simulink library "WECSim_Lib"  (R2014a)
settings: Solver=ode45  StartTime=0.0  StopTime=10.0  RelTol=1e-3
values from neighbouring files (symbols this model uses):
  geometry = 'NOT DEFINED'    [bodyClass.m]
  m = plot(Rel.WEC_Sim_org.time(find(Rel.WEC_Sim_org.time==350):end),     Rel.WEC_Sim_org.heave(find(Rel.WEC_Sim_org.time==350):end),'r-',     Rel.WEC_Sim_new.time(find(Rel.WEC_Sim_new.time==350):end),     Rel.WEC_Sim_new.heave(find(Rel.WEC_Sim_new.time==350):end),'k-')    [runTestCase.m]
  simu = simulationClass    [wecSim.m]
  waves = waveClass(waves.type,0,0,simu,'Imported',waves.randPreDefined,waves.spectrumDataFile)    [waveSetup.m]
undefined symbols (not defined in the file or in its folder): body, constraint, deg, flap, kg, N, pto, rad, s, X, Y, Z
libraries: nesl_utility x41, sm_lib x30
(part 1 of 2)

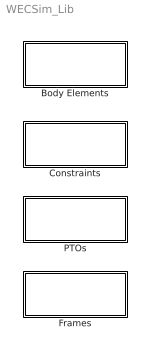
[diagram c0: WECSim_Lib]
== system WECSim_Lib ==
  Body Elements : Subsystem
  Constraints : Subsystem
  Frames : Subsystem
  PTOs : Subsystem

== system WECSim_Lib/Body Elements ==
  Rigid Body : Subsystem

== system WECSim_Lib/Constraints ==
  Fixed : Subsystem
  Floating : Subsystem
  Heave : Subsystem
  Pitch : Subsystem
  Surge : Subsystem

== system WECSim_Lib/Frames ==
  Global Reference Frame : Subsystem

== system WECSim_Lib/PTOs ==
  Rotational PTO (Local RY) : Subsystem
  Translational PTO (Local X) : Subsystem
  Translational PTO (Local Z) : Subsystem

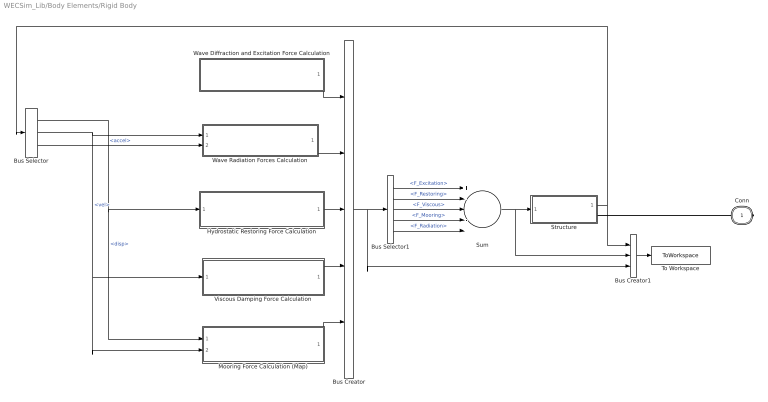
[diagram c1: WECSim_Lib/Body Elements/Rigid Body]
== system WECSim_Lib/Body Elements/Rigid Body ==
  Bus Creator : BusCreator  Inputs=5
  Bus Creator1 : BusCreator  Inputs=3
  Bus Selector : BusSelector  OutputSignals=disp,vel,accel
  Bus Selector1 : BusSelector  OutputSignals=F_Excitation,F_Restoring,F_Viscous,F_Mooring,F_Radiation
  Hydrostatic Restoring Force Calculation : Subsystem
  Mooring Force Calculation (Map) : Subsystem
  Structure : Subsystem
  Sum : Sum  Inputs=+----
  To Workspace : ToWorkspace  VariableName=Flap_out  SaveFormat=Structure With Time  SampleTime=-1
  Viscous Damping Force Calculation : Subsystem
  Wave Diffraction and Excitation Force Calculation : Subsystem
  Wave Radiation Forces Calculation : Subsystem
  Conn : PMIOPort  Port=1  Side=Right
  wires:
  Sum/1 -> Bus Creator1/2, Structure/1(F_vector)
  Bus Selector/1 -> Mooring Force Calculation (Map)/1(Displacement), Hydrostatic Restoring Force Calculation/1(Displacement)  "<disp>"
  Bus Selector/2 -> Mooring Force Calculation (Map)/2(Velocity), Viscous Damping Force Calculation/1(Velocity), Wave Radiation Forces Calculation/1(Velocity)  "<vel>"
  Structure/1(Response) -> Bus Selector/1, Bus Creator1/1
  Bus Creator/1 -> Bus Creator1/3, Bus Selector1/1
  Bus Creator1/1 -> To Workspace/1
  Bus Selector/3 -> Wave Radiation Forces Calculation/2(Acceleration)  "<accel>"
  Mooring Force Calculation (Map)/1(F_Mooring) -> Bus Creator/5
  Viscous Damping Force Calculation/1(F_Viscous) -> Bus Creator/4
  Hydrostatic Restoring Force Calculation/1(F_Restoring) -> Bus Creator/3
  Wave Radiation Forces Calculation/1(F_Radiation) -> Bus Creator/2
  Wave Diffraction and Excitation Force Calculation/1(F_Excitation) -> Bus Creator/1
  Bus Selector1/1 -> Sum/1  "<F_Excitation>"
  Bus Selector1/2 -> Sum/2  "<F_Restoring>"
  Bus Selector1/3 -> Sum/3  "<F_Viscous>"
  Bus Selector1/4 -> Sum/4  "<F_Mooring>"
  Bus Selector1/5 -> Sum/5  "<F_Radiation>"
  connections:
  Structure/RConn1 -- Conn/RConn1

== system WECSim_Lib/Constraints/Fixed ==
  Mux : Mux  Inputs=2
  PSS : nesl_utility/PS-Simulink Converter  PhysicalDomain=network_engine_domain  SubClassName=ps_output  LeftPortType=input  RightPortType=output  PseudoPeriodic=off  Frequencies=[]  Unit=1  AffineConversion=off
  PSS1 : nesl_utility/PS-Simulink Converter  PhysicalDomain=network_engine_domain  SubClassName=ps_output  LeftPortType=input  RightPortType=output  PseudoPeriodic=off  Frequencies=[]  Unit=1  AffineConversion=off
  Weld Joint : sm_lib/Joints/Weld Joint  SenseConstraintForce=on  SenseConstraintForceX=off  SenseConstraintForceY=off  SenseConstraintForceZ=off  SenseConstraintTorque=on  SenseConstraintTorqueX=off  SenseConstraintTorqueY=off  SenseConstraintTorqueZ=off  SenseTotalForce=off  SenseTotalForceX=off  SenseTotalForceY=off  SenseTotalForceZ=off  SenseTotalTorque=off  SenseTotalTorqueX=off  SenseTotalTorqueY=off  SenseTotalTorqueZ=off  CompositeWrenchDir=FollowerOnBase  CompositeWrenchFrame=BaseFrame  BlockFunction=simmechanics.library.joints.weld_joint
  output : ToWorkspace  VariableName=constraint1_out  SaveFormat=Structure With Time  SampleTime=-1
  B : PMIOPort  Port=1  Side=Left
  F : PMIOPort  Port=2  Side=Right
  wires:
  PSS/1 -> Mux/1
  PSS1/1 -> Mux/2
  Mux/1 -> output/1  "Constraint Forces"
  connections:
  Weld Joint/LConn1 -- B/RConn1
  F/RConn1 -- Weld Joint/RConn1
  PSS1/LConn1 -- Weld Joint/RConn3
  PSS/LConn1 -- Weld Joint/RConn2

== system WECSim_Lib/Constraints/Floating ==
  Mux : Mux  Inputs=2
  PSS : nesl_utility/PS-Simulink Converter  PhysicalDomain=network_engine_domain  SubClassName=ps_output  LeftPortType=input  RightPortType=output  PseudoPeriodic=off  Frequencies=[]  Unit=1  AffineConversion=off
  PSS1 : nesl_utility/PS-Simulink Converter  PhysicalDomain=network_engine_domain  SubClassName=ps_output  LeftPortType=input  RightPortType=output  PseudoPeriodic=off  Frequencies=[]  Unit=1  AffineConversion=off
  Planar Joint : sm_lib/Joints/Planar Joint  SenseConstraintForce=on  SenseConstraintForceX=off  SenseConstraintForceY=off  SenseConstraintForceZ=off  SenseConstraintTorque=on  SenseConstraintTorqueX=off  SenseConstraintTorqueY=off  SenseConstraintTorqueZ=off  SenseTotalForce=off  SenseTotalForceX=off  SenseTotalForceY=off  SenseTotalForceZ=off  SenseTotalTorque=off  SenseTotalTorqueX=off  SenseTotalTorqueY=off  SenseTotalTorqueZ=off  CompositeWrenchDir=FollowerOnBase  CompositeWrenchFrame=BaseFrame  PxEquilibriumPosition=0  PxEquilibriumPositionUnits=m  PxSpringStiffness=0  PxSpringStiffnessUnits=N/m  PxDampingCoefficient=0  PxDampingCoefficientUnits=N/(m/s)  PxTorqueActuationMode=NoTorque  PxMotionActuationMode=ComputedMotion  PxSensePosition=off  PxSenseVelocity=off  PxSenseAcceleration=off  PxSenseTorqueForce=off  PxPositionTargetValue=0  PxPositionTargetValueUnits=m  PxPositionTargetSpecify=off  PxPositionTargetPriority=High  PxVelocityTargetValue=0  PxVelocityTargetValueUnits=m/s  PxVelocityTargetSpecify=off  PxVelocityTargetPriority=High  PyEquilibriumPosition=0  PyEquilibriumPositionUnits=m  PySpringStiffness=0  PySpringStiffnessUnits=N/m  PyDampingCoefficient=0  PyDampingCoefficientUnits=N/(m/s)  PyTorqueActuationMode=NoTorque  PyMotionActuationMode=ComputedMotion  PySensePosition=off  PySenseVelocity=off  PySenseAcceleration=off  PySenseTorqueForce=off  PyPositionTargetValue=0  PyPositionTargetValueUnits=m  PyPositionTargetSpecify=off  PyPositionTargetPriority=High  PyVelocityTargetValue=0  PyVelocityTargetValueUnits=m/s  PyVelocityTargetSpecify=off  PyVelocityTargetPriority=High  RzEquilibriumPosition=0  RzEquilibriumPositionUnits=deg  RzSpringStiffness=0  RzSpringStiffnessUnits=N*m/deg  RzDampingCoefficient=0  RzDampingCoefficientUnits=N*m/(deg/s)  RzTorqueActuationMode=NoTorque  RzMotionActuationMode=ComputedMotion  RzSensePosition=off  RzSenseVelocity=off  RzSenseAcceleration=off  RzSenseTorqueForce=off  RzPositionTargetValue=0  RzPositionTargetValueUnits=deg  RzPositionTargetSpecify=off  RzPositionTargetPriority=High  RzVelocityTargetValue=0  RzVelocityTargetValueUnits=deg/s  RzVelocityTargetSpecify=off  RzVelocityTargetPriority=High  BlockFunction=simmechanics.library.joints.planar_joint
  Rigid Transform : sm_lib/Frames and Transforms/Rigid Transform  TranslationMethod=Cartesian  TranslationLengthUnit=m  TranslationStandardAxis=+Z  TranslationStandardOffset=0  TranslationCartesianOffset=[0 0 0]  TranslationROffset=0  TranslationROffsetUnits=m  TranslationZOffset=0  TranslationZOffsetUnits=m  TranslationThetaOffset=0  TranslationThetaOffsetUnits=deg  RotationMethod=StandardAxis  RotationAngleUnits=deg  RotationStandardAxis=+X  RotationAngle=90  RotationArbitraryAxis=[0 0 1]  FollAlignAxisA=+X  BaseAlignAxisA=+Y  FollAlignAxisB=+Y  BaseAlignAxisB=+Z  BlockFunction=simmechanics.library.frames_transforms.rigid_transform
  Rigid Transform1 : sm_lib/Frames and Transforms/Rigid Transform  TranslationMethod=Cartesian  TranslationLengthUnit=m  TranslationStandardAxis=+Z  TranslationStandardOffset=0  TranslationCartesianOffset=[0 0 0]  TranslationROffset=0  TranslationROffsetUnits=m  TranslationZOffset=0  TranslationZOffsetUnits=m  TranslationThetaOffset=0  TranslationThetaOffsetUnits=deg  RotationMethod=StandardAxis  RotationAngleUnits=deg  RotationStandardAxis=+X  RotationAngle=90  RotationArbitraryAxis=[0 0 1]  FollAlignAxisA=+X  BaseAlignAxisA=+Y  FollAlignAxisB=+Y  BaseAlignAxisB=+Z  BlockFunction=simmechanics.library.frames_transforms.rigid_transform
  output : ToWorkspace  VariableName=constraint1_out  SaveFormat=Structure With Time  SampleTime=-1
  B : PMIOPort  Port=1  Side=Left
  F : PMIOPort  Port=2  Side=Right
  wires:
  PSS/1 -> Mux/1
  PSS1/1 -> Mux/2
  Mux/1 -> output/1  "Constraint Forces"
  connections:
  Rigid Transform1/LConn1 -- F/RConn1
  Planar Joint/RConn1 -- Rigid Transform1/RConn1
  Rigid Transform/RConn1 -- Planar Joint/LConn1
  B/RConn1 -- Rigid Transform/LConn1
  PSS/LConn1 -- Planar Joint/RConn2
  PSS1/LConn1 -- Planar Joint/RConn3

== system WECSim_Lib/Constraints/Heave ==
  Mux : Mux  Inputs=2
  PSS : nesl_utility/PS-Simulink Converter  PhysicalDomain=network_engine_domain  SubClassName=ps_output  LeftPortType=input  RightPortType=output  PseudoPeriodic=off  Frequencies=[]  Unit=1  AffineConversion=off
  PSS1 : nesl_utility/PS-Simulink Converter  PhysicalDomain=network_engine_domain  SubClassName=ps_output  LeftPortType=input  RightPortType=output  PseudoPeriodic=off  Frequencies=[]  Unit=1  AffineConversion=off
  Translational Constraint (Prismatic Joint) : sm_lib/Joints/Prismatic Joint  SenseConstraintForce=on  SenseConstraintForceX=off  SenseConstraintForceY=off  SenseConstraintForceZ=off  SenseConstraintTorque=on  SenseConstraintTorqueX=off  SenseConstraintTorqueY=off  SenseConstraintTorqueZ=off  SenseTotalForce=off  SenseTotalForceX=off  SenseTotalForceY=off  SenseTotalForceZ=off  SenseTotalTorque=off  SenseTotalTorqueX=off  SenseTotalTorqueY=off  SenseTotalTorqueZ=off  CompositeWrenchDir=FollowerOnBase  CompositeWrenchFrame=BaseFrame  EquilibriumPosition=0  EquilibriumPositionUnits=m  SpringStiffness=0  SpringStiffnessUnits=N/m  DampingCoefficient=0  DampingCoefficientUnits=N/(m/s)  TorqueActuationMode=NoTorque  MotionActuationMode=ComputedMotion  SensePosition=off  SenseVelocity=off  SenseAcceleration=off  SenseTorqueForce=off  PositionTargetValue=0  PositionTargetValueUnits=m  PositionTargetSpecify=off  PositionTargetPriority=High  VelocityTargetValue=0  VelocityTargetValueUnits=m/s  VelocityTargetSpecify=off  VelocityTargetPriority=High  BlockFunction=simmechanics.library.joints.prismatic_joint
  output : ToWorkspace  VariableName=constraint1_out  SaveFormat=Structure With Time  SampleTime=-1
  F : PMIOPort  Port=1  Side=Right
  B : PMIOPort  Port=2  Side=Left
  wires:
  PSS/1 -> Mux/1
  PSS1/1 -> Mux/2
  Mux/1 -> output/1  "Constraint Forces"
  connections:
  B/RConn1 -- Translational Constraint (Prismatic Joint)/LConn1
  Translational Constraint (Prismatic Joint)/RConn1 -- F/RConn1
  PSS/LConn1 -- Translational Constraint (Prismatic Joint)/RConn2
  PSS1/LConn1 -- Translational Constraint (Prismatic Joint)/RConn3

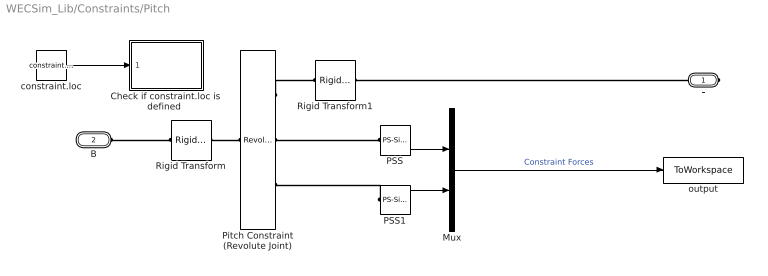
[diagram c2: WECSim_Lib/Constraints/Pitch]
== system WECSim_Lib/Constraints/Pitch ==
  "Check if constraint.loc is defined " : MATLAB Function  TreatAsAtomicUnit=on
  Mux : Mux  Inputs=2
  PSS : nesl_utility/PS-Simulink Converter  PhysicalDomain=network_engine_domain  SubClassName=ps_output  LeftPortType=input  RightPortType=output  PseudoPeriodic=off  Frequencies=[]  Unit=1  AffineConversion=off
  PSS1 : nesl_utility/PS-Simulink Converter  PhysicalDomain=network_engine_domain  SubClassName=ps_output  LeftPortType=input  RightPortType=output  PseudoPeriodic=off  Frequencies=[]  Unit=1  AffineConversion=off
  Pitch Constraint (Revolute Joint) : sm_lib/Joints/Revolute Joint  SenseConstraintForce=on  SenseConstraintForceX=off  SenseConstraintForceY=off  SenseConstraintForceZ=off  SenseConstraintTorque=on  SenseConstraintTorqueX=off  SenseConstraintTorqueY=off  SenseConstraintTorqueZ=off  SenseTotalForce=off  SenseTotalForceX=off  SenseTotalForceY=off  SenseTotalForceZ=off  SenseTotalTorque=off  SenseTotalTorqueX=off  SenseTotalTorqueY=off  SenseTotalTorqueZ=off  CompositeWrenchDir=FollowerOnBase  CompositeWrenchFrame=BaseFrame  EquilibriumPosition=0  EquilibriumPositionUnits=deg  SpringStiffness=0  SpringStiffnessUnits=N*m/deg  DampingCoefficient=0  DampingCoefficientUnits=N*m/(rad/s)  TorqueActuationMode=NoTorque  MotionActuationMode=ComputedMotion  SensePosition=off  SenseVelocity=off  SenseAcceleration=off  SenseTorqueForce=off  PositionTargetValue=0  PositionTargetValueUnits=deg  PositionTargetSpecify=off  PositionTargetPriority=High  VelocityTargetValue=0  VelocityTargetValueUnits=deg/s  VelocityTargetSpecify=off  VelocityTargetPriority=High  BlockFunction=simmechanics.library.joints.revolute_joint
  Rigid Transform : sm_lib/Frames and Transforms/Rigid Transform  TranslationMethod=Cartesian  TranslationLengthUnit=m  TranslationStandardAxis=+Z  TranslationStandardOffset=0  TranslationCartesianOffset=constraint.loc  TranslationROffset=0  TranslationROffsetUnits=m  TranslationZOffset=0  TranslationZOffsetUnits=m  TranslationThetaOffset=0  TranslationThetaOffsetUnits=deg  RotationMethod=StandardAxis  RotationAngleUnits=deg  RotationStandardAxis=+X  RotationAngle=90  RotationArbitraryAxis=[0 0 1]  FollAlignAxisA=+X  BaseAlignAxisA=+Y  FollAlignAxisB=+Y  BaseAlignAxisB=+Z  BlockFunction=simmechanics.library.frames_transforms.rigid_transform
  Rigid Transform1 : sm_lib/Frames and Transforms/Rigid Transform  TranslationMethod=Cartesian  TranslationLengthUnit=m  TranslationStandardAxis=+Z  TranslationStandardOffset=0  TranslationCartesianOffset=constraint.loc  TranslationROffset=0  TranslationROffsetUnits=m  TranslationZOffset=0  TranslationZOffsetUnits=m  TranslationThetaOffset=0  TranslationThetaOffsetUnits=deg  RotationMethod=StandardAxis  RotationAngleUnits=deg  RotationStandardAxis=+X  RotationAngle=90  RotationArbitraryAxis=[0 0 1]  FollAlignAxisA=+X  BaseAlignAxisA=+Y  FollAlignAxisB=+Y  BaseAlignAxisB=+Z  BlockFunction=simmechanics.library.frames_transforms.rigid_transform
  constraint.loc : Constant  Value=constraint.loc(1)  VectorParams1D=off
  output : ToWorkspace  VariableName=constraint1_out  SaveFormat=Structure With Time  SampleTime=-1
  F : PMIOPort  Port=1  Side=Right
  B : PMIOPort  Port=2  Side=Left
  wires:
  PSS/1 -> Mux/1
  PSS1/1 -> Mux/2
  Mux/1 -> output/1  "Constraint Forces"
  constraint.loc/1 -> "Check if constraint.loc is defined "/1(u)
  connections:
  Pitch Constraint (Revolute Joint)/LConn1 -- Rigid Transform/RConn1
  Pitch Constraint (Revolute Joint)/RConn1 -- Rigid Transform1/RConn1
  B/RConn1 -- Rigid Transform/LConn1
  F/RConn1 -- Rigid Transform1/LConn1
  PSS/LConn1 -- Pitch Constraint (Revolute Joint)/RConn2
  PSS1/LConn1 -- Pitch Constraint (Revolute Joint)/RConn3

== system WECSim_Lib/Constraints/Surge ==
  Mux : Mux  Inputs=2
  PSS : nesl_utility/PS-Simulink Converter  PhysicalDomain=network_engine_domain  SubClassName=ps_output  LeftPortType=input  RightPortType=output  PseudoPeriodic=off  Frequencies=[]  Unit=1  AffineConversion=off
  PSS1 : nesl_utility/PS-Simulink Converter  PhysicalDomain=network_engine_domain  SubClassName=ps_output  LeftPortType=input  RightPortType=output  PseudoPeriodic=off  Frequencies=[]  Unit=1  AffineConversion=off
  Rigid Transform : sm_lib/Frames and Transforms/Rigid Transform  TranslationMethod=None  TranslationLengthUnit=m  TranslationStandardAxis=+Z  TranslationStandardOffset=0  TranslationCartesianOffset=[0 0 0]  TranslationROffset=0  TranslationROffsetUnits=m  TranslationZOffset=0  TranslationZOffsetUnits=m  TranslationThetaOffset=0  TranslationThetaOffsetUnits=deg  RotationMethod=StandardAxis  RotationAngleUnits=deg  RotationStandardAxis=+Y  RotationAngle=90  RotationArbitraryAxis=[0 0 1]  FollAlignAxisA=+X  BaseAlignAxisA=+Y  FollAlignAxisB=+Y  BaseAlignAxisB=+Z  BlockFunction=simmechanics.library.frames_transforms.rigid_transform
  Rigid Transform1 : sm_lib/Frames and Transforms/Rigid Transform  TranslationMethod=None  TranslationLengthUnit=m  TranslationStandardAxis=+Z  TranslationStandardOffset=0  TranslationCartesianOffset=[0 0 0]  TranslationROffset=0  TranslationROffsetUnits=m  TranslationZOffset=0  TranslationZOffsetUnits=m  TranslationThetaOffset=0  TranslationThetaOffsetUnits=deg  RotationMethod=StandardAxis  RotationAngleUnits=deg  RotationStandardAxis=+Y  RotationAngle=90  RotationArbitraryAxis=[0 0 1]  FollAlignAxisA=+X  BaseAlignAxisA=+Y  FollAlignAxisB=+Y  BaseAlignAxisB=+Z  BlockFunction=simmechanics.library.frames_transforms.rigid_transform
  Translational Constraint (Prismatic Joint) : sm_lib/Joints/Prismatic Joint  SenseConstraintForce=on  SenseConstraintForceX=off  SenseConstraintForceY=off  SenseConstraintForceZ=off  SenseConstraintTorque=on  SenseConstraintTorqueX=off  SenseConstraintTorqueY=off  SenseConstraintTorqueZ=off  SenseTotalForce=off  SenseTotalForceX=off  SenseTotalForceY=off  SenseTotalForceZ=off  SenseTotalTorque=off  SenseTotalTorqueX=off  SenseTotalTorqueY=off  SenseTotalTorqueZ=off  CompositeWrenchDir=FollowerOnBase  CompositeWrenchFrame=BaseFrame  EquilibriumPosition=0  EquilibriumPositionUnits=m  SpringStiffness=0  SpringStiffnessUnits=N/m  DampingCoefficient=0  DampingCoefficientUnits=N/(m/s)  TorqueActuationMode=NoTorque  MotionActuationMode=ComputedMotion  SensePosition=off  SenseVelocity=off  SenseAcceleration=off  SenseTorqueForce=off  PositionTargetValue=0  PositionTargetValueUnits=m  PositionTargetSpecify=off  PositionTargetPriority=High  VelocityTargetValue=0  VelocityTargetValueUnits=m/s  VelocityTargetSpecify=off  VelocityTargetPriority=High  BlockFunction=simmechanics.library.joints.prismatic_joint
  output : ToWorkspace  VariableName=constraint1_out  SaveFormat=Structure With Time  SampleTime=-1
  F : PMIOPort  Port=1  Side=Right
  B : PMIOPort  Port=2  Side=Left
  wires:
  PSS/1 -> Mux/1
  PSS1/1 -> Mux/2
  Mux/1 -> output/1  "Constraint Forces"
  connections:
  Rigid Transform1/LConn1 -- F/RConn1
  Rigid Transform1/RConn1 -- Translational Constraint (Prismatic Joint)/RConn1
  Rigid Transform/RConn1 -- Translational Constraint (Prismatic Joint)/LConn1
  Rigid Transform/LConn1 -- B/RConn1
  PSS/LConn1 -- Translational Constraint (Prismatic Joint)/RConn2
  PSS1/LConn1 -- Translational Constraint (Prismatic Joint)/RConn3

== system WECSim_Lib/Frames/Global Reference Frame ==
  note: NOTE:Must be a fixed time step solver changed to ode4 (fixed step)
  Clock : Clock
  Mean Free Surface : sm_lib/Body Elements/Solid  InertiaType=Custom  Mass=10^20  MassUnits=kg  CenterOfMass=[0 0 0]  CenterOfMassUnits=m  MomentsOfInertia=[10^20 10^20 10^20]  MomentsOfInertiaUnits=kg*m^2  ProductsOfInertia=[0 0 0]  ProductsOfInertiaUnits=kg*m^2  DensityBased=on  Density=1000  DensityUnits=kg/(m^3)  GraphicType=FromGeometry  MarkerShape=Sphere  MarkerSize=10  MarkerSizeUnits=m  GraphicVisPropType=SimpleVisualProperties  GraphicDiffuseColor=[0.0 0.6 0.8]  GraphicSpecularColor=[0.5 0.5 0.5 1.0]  GraphicAmbientColor=[0.15 0.15 0.15 1.0]  GraphicEmissiveColor=[0.0 0.0 0.0 1.0]  GraphicShininess=75  GraphicOpacity=0.3  GeometryShape=GeneralExtrusion  RectangleSize=[1 1]  RectangleSizeUnits=m  BrickDimensions=[1 1 1]  BrickDimensionUnits=m  CylinderRadius=1  CylinderRadiusUnits=m  CylinderLength=1  CylinderLengthUnits=m  SphereRadius=1  SphereRadiusUnits=m  EllipsoidRadii=[1 1 1]  EllipsoidRadiiUnits=m  ExtrusionCrossSection=[simu.domainSize simu.domainSize; -simu.domainSize simu.domainSize; -simu.domainSize -simu.domainSize; simu.domainSize -simu.domainSize]  ExtrusionCrossSectionUnits=m  ExtrusionLength=simu.domainSize/200  ExtrusionLengthUnits=m  PolygonNumSides=3  PolygonOuterRadius=1  PolygonOuterRadiusUnits=m  ExtGeomFileType=STL  ExtGeomFileUnits=m  RevolutionCrossSection=[1 1; 1 -1; 2 -1; 2 1]  RevolutionCrossSectionUnits=m  RevolutionExtent=Full  RevolutionAngle=180  RevolutionAngleUnits=deg  BlockFunction=simmechanics.library.body_elements.solid
  Mechanism Configuration1 : sm_lib/Utilities/Mechanism Configuration  UniformGravity=Constant  GravityVector=[0 0 0]  GravityUnits=m/s^2  LinearizationDelta=0.001  BlockFunction=simmechanics.library.utilities.mechanism_configuration
  Rigid Transform : sm_lib/Frames and Transforms/Rigid Transform  TranslationMethod=Cartesian  TranslationLengthUnit=m  TranslationStandardAxis=+Z  TranslationStandardOffset=0  TranslationCartesianOffset=[0 0 -waves.waterDepth]  TranslationROffset=0  TranslationROffsetUnits=m  TranslationZOffset=0  TranslationZOffsetUnits=m  TranslationThetaOffset=0  TranslationThetaOffsetUnits=deg  RotationMethod=None  RotationAngleUnits=deg  RotationStandardAxis=+Z  RotationAngle=0  RotationArbitraryAxis=[0 0 1]  FollAlignAxisA=+X  BaseAlignAxisA=+Y  FollAlignAxisB=+Y  BaseAlignAxisB=+Z  BlockFunction=simmechanics.library.frames_transforms.rigid_transform
  Seabed : sm_lib/Body Elements/Solid  InertiaType=Custom  Mass=10^20  MassUnits=kg  CenterOfMass=[0 0 0]  CenterOfMassUnits=m  MomentsOfInertia=[10^20 10^20 10^20]  MomentsOfInertiaUnits=kg*m^2  ProductsOfInertia=[0 0 0]  ProductsOfInertiaUnits=kg*m^2  DensityBased=on  Density=1000  DensityUnits=kg/(m^3)  GraphicType=FromGeometry  MarkerShape=Sphere  MarkerSize=10  MarkerSizeUnits=m  GraphicVisPropType=SimpleVisualProperties  GraphicDiffuseColor=[0.4 0.4 0.0]  GraphicSpecularColor=[0.5 0.5 0.5 1.0]  GraphicAmbientColor=[0.15 0.15 0.15 1.0]  GraphicEmissiveColor=[0.0 0.0 0.0 1.0]  GraphicShininess=75  GraphicOpacity=1  GeometryShape=GeneralExtrusion  RectangleSize=[1 1]  RectangleSizeUnits=m  BrickDimensions=[1 1 1]  BrickDimensionUnits=m  CylinderRadius=1  CylinderRadiusUnits=m  CylinderLength=1  CylinderLengthUnits=m  SphereRadius=1  SphereRadiusUnits=m  EllipsoidRadii=[1 1 1]  EllipsoidRadiiUnits=m  ExtrusionCrossSection=[simu.domainSize simu.domainSize; -simu.domainSize simu.domainSize; -simu.domainSize -simu.domainSize; simu.domainSize -simu.domainSize]  ExtrusionCrossSectionUnits=m  ExtrusionLength=simu.domainSize/100  ExtrusionLengthUnits=m  PolygonNumSides=3  PolygonOuterRadius=1  PolygonOuterRadiusUnits=m  ExtGeomFileType=STL  ExtGeomFileUnits=m  RevolutionCrossSection=[1 1; 1 -1; 2 -1; 2 1]  RevolutionCrossSectionUnits=m  RevolutionExtent=Full  RevolutionAngle=180  RevolutionAngleUnits=deg  BlockFunction=simmechanics.library.body_elements.solid
  Solver Configuration : nesl_utility/Solver Configuration  PhysicalDomain=network_engine_domain  SubClassName=solver  LeftPortType=input  RightPortType=generic  Accelerate=off  Tones=[]  Harmonics=[]  SimulateNoise=off  Profile=off  UseLocalSampling=off  EnableSwitchedLinearOptims=on  FrequencyDomain=off  UseCCode=off  RelTol=0.001  AbsTol=1e-06  MinStep=1e-09  ToWorkspace=off  DoDC=on  ResidualTolerance=1e-9  UseLocalSolver=off  LocalSolverChoice=NE_BACKWARD_EULER_ADVANCER  LocalSolverSampleTime=.001  DoFixedCost=off  MaxNonlinIter=3  MaxModeIter=2  LinearAlgebra=Sparse  DelaysMemoryBudget=1024  AutomaticFiltering=on  FilteringTimeConstant=0.001
  World Frame2 : sm_lib/Frames and Transforms/World Frame  BlockFunction=simmechanics.library.frames_transforms.world_frame
  Conn : PMIOPort  Port=1  Side=Right
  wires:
  Clock/1 -> [Clock]
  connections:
  Mechanism Configuration1/RConn1 -- World Frame2/RConn1 -- Solver Configuration/RConn1 -- Mean Free Surface/RConn1 -- Rigid Transform/LConn1 -- Conn/RConn1
  Seabed/RConn1 -- Rigid Transform/RConn1

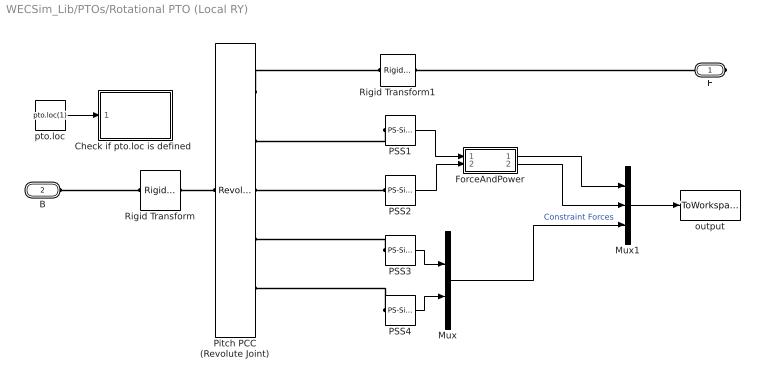
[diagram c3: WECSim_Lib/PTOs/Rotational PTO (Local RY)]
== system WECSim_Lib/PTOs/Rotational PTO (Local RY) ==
  "Check if pto.loc is defined " : MATLAB Function  TreatAsAtomicUnit=on
  ForceAndPower : Subsystem
  Mux : Mux  Inputs=2
  Mux1 : Mux  Inputs=3
  PSS{1..4} (4 alike) : nesl_utility/PS-Simulink Converter  PhysicalDomain=network_engine_domain  SubClassName=ps_output  LeftPortType=input  RightPortType=output  PseudoPeriodic=off  Frequencies=[]  Unit=1  AffineConversion=off
  Pitch PCC (Revolute Joint) : sm_lib/Joints/Revolute Joint  SenseConstraintForce=on  SenseConstraintForceX=off  SenseConstraintForceY=off  SenseConstraintForceZ=off  SenseConstraintTorque=on  SenseConstraintTorqueX=off  SenseConstraintTorqueY=off  SenseConstraintTorqueZ=off  SenseTotalForce=off  SenseTotalForceX=off  SenseTotalForceY=off  SenseTotalForceZ=off  SenseTotalTorque=off  SenseTotalTorqueX=off  SenseTotalTorqueY=off  SenseTotalTorqueZ=off  CompositeWrenchDir=FollowerOnBase  CompositeWrenchFrame=BaseFrame  EquilibriumPosition=0  EquilibriumPositionUnits=deg  SpringStiffness=pto.k  SpringStiffnessUnits=N*m/rad  DampingCoefficient=pto.c  DampingCoefficientUnits=N*m/(rad/s)  TorqueActuationMode=NoTorque  MotionActuationMode=ComputedMotion  SensePosition=on  SenseVelocity=on  SenseAcceleration=off  SenseTorqueForce=off  PositionTargetValue=0  PositionTargetValueUnits=deg  PositionTargetSpecify=off  PositionTargetPriority=High  VelocityTargetValue=0  VelocityTargetValueUnits=deg/s  VelocityTargetSpecify=off  VelocityTargetPriority=High  BlockFunction=simmechanics.library.joints.revolute_joint
  Rigid Transform : sm_lib/Frames and Transforms/Rigid Transform  TranslationMethod=Cartesian  TranslationLengthUnit=m  TranslationStandardAxis=+Z  TranslationStandardOffset=0  TranslationCartesianOffset=pto.loc  TranslationROffset=0  TranslationROffsetUnits=m  TranslationZOffset=0  TranslationZOffsetUnits=m  TranslationThetaOffset=0  TranslationThetaOffsetUnits=deg  RotationMethod=StandardAxis  RotationAngleUnits=deg  RotationStandardAxis=+X  RotationAngle=90  RotationArbitraryAxis=[0 0 1]  FollAlignAxisA=+X  BaseAlignAxisA=+Y  FollAlignAxisB=+Y  BaseAlignAxisB=+Z  BlockFunction=simmechanics.library.frames_transforms.rigid_transform
  Rigid Transform1 : sm_lib/Frames and Transforms/Rigid Transform  TranslationMethod=Cartesian  TranslationLengthUnit=m  TranslationStandardAxis=+Z  TranslationStandardOffset=0  TranslationCartesianOffset=pto.loc  TranslationROffset=0  TranslationROffsetUnits=m  TranslationZOffset=0  TranslationZOffsetUnits=m  TranslationThetaOffset=0  TranslationThetaOffsetUnits=deg  RotationMethod=StandardAxis  RotationAngleUnits=deg  RotationStandardAxis=+X  RotationAngle=90  RotationArbitraryAxis=[0 0 1]  FollAlignAxisA=+X  BaseAlignAxisA=+Y  FollAlignAxisB=+Y  BaseAlignAxisB=+Z  BlockFunction=simmechanics.library.frames_transforms.rigid_transform
  output : ToWorkspace  VariableName=Joint1_out  SaveFormat=Structure With Time  SampleTime=-1
  pto.loc : Constant  Value=pto.loc(1)  VectorParams1D=off
  F : PMIOPort  Port=1  Side=Right
  B : PMIOPort  Port=2  Side=Left
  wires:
  PSS2/1 -> ForceAndPower/2(Vel)
  PSS1/1 -> ForceAndPower/1(Pos)
  PSS3/1 -> Mux/1
  PSS4/1 -> Mux/2
  Mux/1 -> Mux1/3  "Constraint Forces"
  Mux1/1 -> output/1
  ForceAndPower/1(Force/Torque) -> Mux1/1
  ForceAndPower/2(Power) -> Mux1/2
  pto.loc/1 -> "Check if pto.loc is defined "/1(u)
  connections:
  F/RConn1 -- Rigid Transform1/LConn1
  B/RConn1 -- Rigid Transform/LConn1
  Pitch PCC (Revolute Joint)/RConn1 -- Rigid Transform1/RConn1
  Pitch PCC (Revolute Joint)/LConn1 -- Rigid Transform/RConn1
  PSS2/LConn1 -- Pitch PCC (Revolute Joint)/RConn3
  PSS3/LConn1 -- Pitch PCC (Revolute Joint)/RConn4
  PSS1/LConn1 -- Pitch PCC (Revolute Joint)/RConn2
  PSS4/LConn1 -- Pitch PCC (Revolute Joint)/RConn5

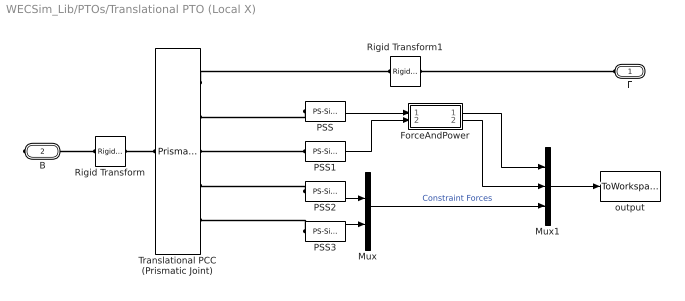
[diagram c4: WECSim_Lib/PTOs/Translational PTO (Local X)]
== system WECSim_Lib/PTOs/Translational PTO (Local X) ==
  ForceAndPower : Subsystem
  Mux : Mux  Inputs=2
  Mux1 : Mux  Inputs=3
  PSS{,1..3} (4 alike) : nesl_utility/PS-Simulink Converter  PhysicalDomain=network_engine_domain  SubClassName=ps_output  LeftPortType=input  RightPortType=output  PseudoPeriodic=off  Frequencies=[]  Unit=1  AffineConversion=off
  Rigid Transform : sm_lib/Frames and Transforms/Rigid Transform  TranslationMethod=None  TranslationLengthUnit=m  TranslationStandardAxis=+Z  TranslationStandardOffset=0  TranslationCartesianOffset=[0 0 0]  TranslationROffset=0  TranslationROffsetUnits=m  TranslationZOffset=0  TranslationZOffsetUnits=m  TranslationThetaOffset=0  TranslationThetaOffsetUnits=deg  RotationMethod=StandardAxis  RotationAngleUnits=deg  RotationStandardAxis=+Y  RotationAngle=90  RotationArbitraryAxis=[0 0 1]  FollAlignAxisA=+X  BaseAlignAxisA=+Y  FollAlignAxisB=+Y  BaseAlignAxisB=+Z  BlockFunction=simmechanics.library.frames_transforms.rigid_transform
  Rigid Transform1 : sm_lib/Frames and Transforms/Rigid Transform  TranslationMethod=None  TranslationLengthUnit=m  TranslationStandardAxis=+Z  TranslationStandardOffset=0  TranslationCartesianOffset=[0 0 0]  TranslationROffset=0  TranslationROffsetUnits=m  TranslationZOffset=0  TranslationZOffsetUnits=m  TranslationThetaOffset=0  TranslationThetaOffsetUnits=deg  RotationMethod=StandardAxis  RotationAngleUnits=deg  RotationStandardAxis=+Y  RotationAngle=90  RotationArbitraryAxis=[0 0 1]  FollAlignAxisA=+X  BaseAlignAxisA=+Y  FollAlignAxisB=+Y  BaseAlignAxisB=+Z  BlockFunction=simmechanics.library.frames_transforms.rigid_transform
  Translational PCC (Prismatic Joint) : sm_lib/Joints/Prismatic Joint  SenseConstraintForce=on  SenseConstraintForceX=off  SenseConstraintForceY=off  SenseConstraintForceZ=off  SenseConstraintTorque=on  SenseConstraintTorqueX=off  SenseConstraintTorqueY=off  SenseConstraintTorqueZ=off  SenseTotalForce=off  SenseTotalForceX=off  SenseTotalForceY=off  SenseTotalForceZ=off  SenseTotalTorque=off  SenseTotalTorqueX=off  SenseTotalTorqueY=off  SenseTotalTorqueZ=off  CompositeWrenchDir=FollowerOnBase  CompositeWrenchFrame=BaseFrame  EquilibriumPosition=0  EquilibriumPositionUnits=m  SpringStiffness=pto.k  SpringStiffnessUnits=N/m  DampingCoefficient=pto.c  DampingCoefficientUnits=N/(m/s)  TorqueActuationMode=NoTorque  MotionActuationMode=ComputedMotion  SensePosition=on  SenseVelocity=on  SenseAcceleration=off  SenseTorqueForce=off  PositionTargetValue=0  PositionTargetValueUnits=m  PositionTargetSpecify=off  PositionTargetPriority=High  VelocityTargetValue=0  VelocityTargetValueUnits=m/s  VelocityTargetSpecify=off  VelocityTargetPriority=High  BlockFunction=simmechanics.library.joints.prismatic_joint
  output : ToWorkspace  VariableName=Joint1_out  SaveFormat=Structure With Time  SampleTime=-1
  F : PMIOPort  Port=1  Side=Left
  B : PMIOPort  Port=2  Side=Right
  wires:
  PSS1/1 -> ForceAndPower/2(Vel)
  PSS2/1 -> Mux/1
  PSS3/1 -> Mux/2
  Mux/1 -> Mux1/3  "Constraint Forces"
  Mux1/1 -> output/1
  ForceAndPower/1(Force) -> Mux1/1
  ForceAndPower/2(Power) -> Mux1/2
  PSS/1 -> ForceAndPower/1(Pos)
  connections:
  Rigid Transform/LConn1 -- B/RConn1
  Rigid Transform/RConn1 -- Translational PCC (Prismatic Joint)/LConn1
  Translational PCC (Prismatic Joint)/RConn1 -- Rigid Transform1/RConn1
  Rigid Transform1/LConn1 -- F/RConn1
  PSS/LConn1 -- Translational PCC (Prismatic Joint)/RConn2
  PSS1/LConn1 -- Translational PCC (Prismatic Joint)/RConn3
  PSS2/LConn1 -- Translational PCC (Prismatic Joint)/RConn4
  PSS3/LConn1 -- Translational PCC (Prismatic Joint)/RConn5

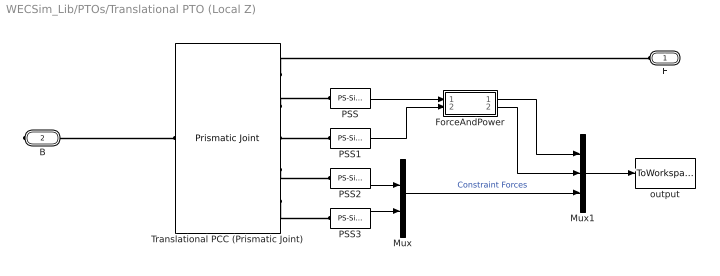
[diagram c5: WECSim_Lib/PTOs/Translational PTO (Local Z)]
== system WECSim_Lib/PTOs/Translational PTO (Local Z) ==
  ForceAndPower : Subsystem
  Mux : Mux  Inputs=2
  Mux1 : Mux  Inputs=3
  PSS{,1..3} (4 alike) : nesl_utility/PS-Simulink Converter  PhysicalDomain=network_engine_domain  SubClassName=ps_output  LeftPortType=input  RightPortType=output  PseudoPeriodic=off  Frequencies=[]  Unit=1  AffineConversion=off
  Translational PCC (Prismatic Joint) : sm_lib/Joints/Prismatic Joint  SenseConstraintForce=on  SenseConstraintForceX=off  SenseConstraintForceY=off  SenseConstraintForceZ=off  SenseConstraintTorque=on  SenseConstraintTorqueX=off  SenseConstraintTorqueY=off  SenseConstraintTorqueZ=off  SenseTotalForce=off  SenseTotalForceX=off  SenseTotalForceY=off  SenseTotalForceZ=off  SenseTotalTorque=off  SenseTotalTorqueX=off  SenseTotalTorqueY=off  SenseTotalTorqueZ=off  CompositeWrenchDir=FollowerOnBase  CompositeWrenchFrame=BaseFrame  EquilibriumPosition=0  EquilibriumPositionUnits=m  SpringStiffness=pto.k  SpringStiffnessUnits=N/m  DampingCoefficient=pto.c  DampingCoefficientUnits=N/(m/s)  TorqueActuationMode=NoTorque  MotionActuationMode=ComputedMotion  SensePosition=on  SenseVelocity=on  SenseAcceleration=off  SenseTorqueForce=off  PositionTargetValue=0  PositionTargetValueUnits=m  PositionTargetSpecify=off  PositionTargetPriority=High  VelocityTargetValue=0  VelocityTargetValueUnits=m/s  VelocityTargetSpecify=off  VelocityTargetPriority=High  BlockFunction=simmechanics.library.joints.prismatic_joint
  output : ToWorkspace  VariableName=Joint1_out  SaveFormat=Structure With Time  SampleTime=-1
  F : PMIOPort  Port=1  Side=Left
  B : PMIOPort  Port=2  Side=Right
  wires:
  PSS1/1 -> ForceAndPower/2(Vel)
  PSS/1 -> ForceAndPower/1(Pos)
  PSS2/1 -> Mux/1
  PSS3/1 -> Mux/2
  Mux/1 -> Mux1/3  "Constraint Forces"
  Mux1/1 -> output/1
  ForceAndPower/1(Force) -> Mux1/1
  ForceAndPower/2(Power) -> Mux1/2
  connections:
  B/RConn1 -- Translational PCC (Prismatic Joint)/LConn1
  Translational PCC (Prismatic Joint)/RConn1 -- F/RConn1
  Translational PCC (Prismatic Joint)/RConn3 -- PSS1/LConn1
  Translational PCC (Prismatic Joint)/RConn2 -- PSS/LConn1
  Translational PCC (Prismatic Joint)/RConn4 -- PSS2/LConn1
  Translational PCC (Prismatic Joint)/RConn5 -- PSS3/LConn1

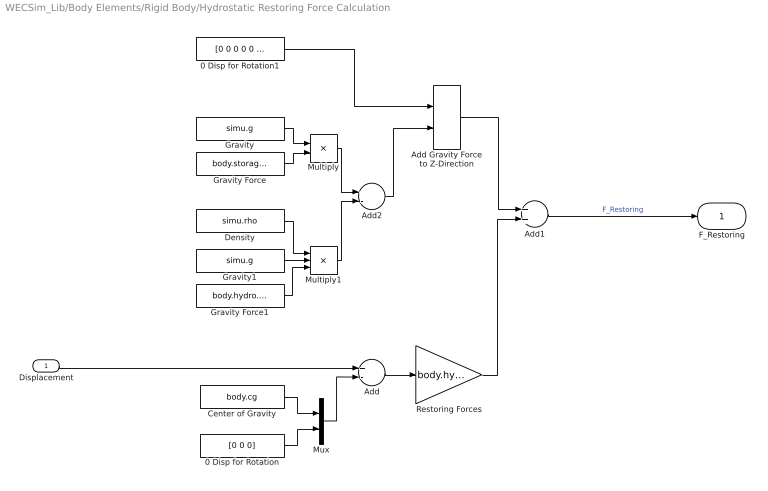
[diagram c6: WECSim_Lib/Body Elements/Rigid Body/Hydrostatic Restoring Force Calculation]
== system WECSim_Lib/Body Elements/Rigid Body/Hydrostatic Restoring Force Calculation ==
  Displacement : Inport
  0 Disp for Rotation : Constant  Value=[0 0 0]
  0 Disp for Rotation1 : Constant  Value=[0 0 0 0 0 0]
  Add : Sum  Inputs=+-
  Add Gravity Force to Z-Direction : Assignment  Indices=3
  Add1 : Sum
  Add2 : Sum  Inputs=+-
  Center of Gravity : Constant  Value=body.cg
  Density : Constant  Value=simu.rho
  Gravity : Constant  Value=simu.g
  Gravity Force : Constant  Value=body.storage.mass
  Gravity Force1 : Constant  Value=body.hydro.data.vol
  Gravity1 : Constant  Value=simu.g
  Multiply : Product  Inputs=**
  Multiply1 : Product  Inputs=***
  Mux : Mux  Inputs=2
  Restoring Forces : Gain  Gain=body.hydroForce.linearHyroRestCoef  Multiplication=Matrix(K*u)
  F_Restoring : Outport
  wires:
  Add/1 -> Restoring Forces/1
  Displacement/1 -> Add/1
  Mux/1 -> Add/2
  Center of Gravity/1 -> Mux/1
  0 Disp for Rotation/1 -> Mux/2
  Gravity/1 -> Multiply/1
  Gravity Force/1 -> Multiply/2
  0 Disp for Rotation1/1 -> Add Gravity Force to Z-Direction/1
  Add Gravity Force to Z-Direction/1 -> Add1/1
  Add1/1 -> F_Restoring/1  "F_Restoring"
  Gravity Force1/1 -> Multiply1/3
  Gravity1/1 -> Multiply1/2
  Density/1 -> Multiply1/1
  Multiply/1 -> Add2/1
  Multiply1/1 -> Add2/2
  Add2/1 -> Add Gravity Force to Z-Direction/2
  Restoring Forces/1 -> Add1/2

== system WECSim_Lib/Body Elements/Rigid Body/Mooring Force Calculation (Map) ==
  Displacement : Inport
  Velocity : Inport  Port=2
  0 Disp for Rotation : Constant  Value=[0 0 0]
  Add : Sum  Inputs=+-
  Center of Gravity : Constant  Value=body.cg
  Mooring Damping : Gain  Gain=body.mooring.c  Multiplication=Matrix(K*u)
  Mooring Stiffness : Gain  Gain=body.mooring.k  Multiplication=Matrix(K*u)
  Mooring Pre-Tension : Constant  Value=body.mooring.preTension
  Mux : Mux  Inputs=2
  sum : Sum  Inputs=++-
  F_Mooring : Outport
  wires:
  Mooring Stiffness/1 -> sum/1
  Velocity/1 -> Mooring Damping/1
  Mooring Damping/1 -> sum/2
  sum/1 -> F_Mooring/1  "F_Mooring"
  Mooring Pre-Tension/1 -> sum/3
  Add/1 -> Mooring Stiffness/1
  Mux/1 -> Add/2
  Displacement/1 -> Add/1
  Center of Gravity/1 -> Mux/1
  0 Disp for Rotation/1 -> Mux/2

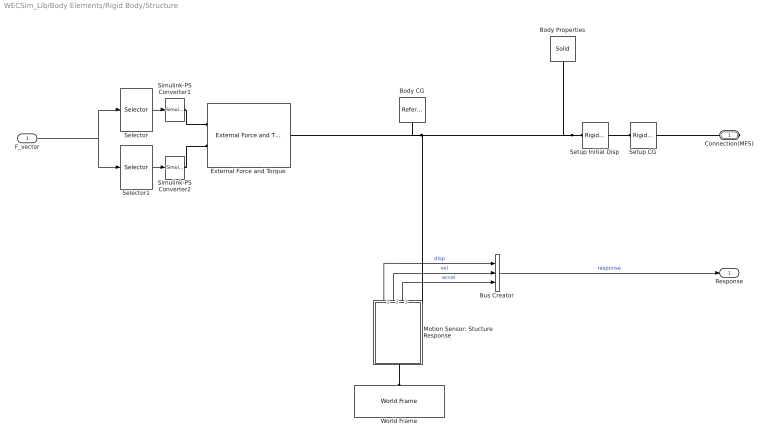
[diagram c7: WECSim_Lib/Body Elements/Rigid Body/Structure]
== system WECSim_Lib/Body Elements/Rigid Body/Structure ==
  F_vector : Inport
  Body CG : sm_lib/Frames and Transforms/Reference Frame  BlockFunction=simmechanics.library.frames_transforms.reference_frame
  Body Properties : sm_lib/Body Elements/Solid  InertiaType=Custom  Mass=body.mass  MassUnits=kg  CenterOfMass=[0 0 0]  CenterOfMassUnits=m  MomentsOfInertia=body.momOfInertia  MomentsOfInertiaUnits=kg*m^2  ProductsOfInertia=[0 0 0]  ProductsOfInertiaUnits=kg*m^2  DensityBased=on  Density=1000  DensityUnits=kg/(m^3)  GraphicType=FromGeometry  MarkerShape=Sphere  MarkerSize=10  MarkerSizeUnits=m  GraphicVisPropType=SimpleVisualProperties  GraphicDiffuseColor=[1 1 0]  GraphicSpecularColor=[0.5 0.5 0.5 1.0]  GraphicAmbientColor=[0.15 0.15 0.15 1.0]  GraphicEmissiveColor=[0.0 0.0 0.0 1.0]  GraphicShininess=75  GraphicOpacity=1  GeometryShape=FromFile  RectangleSize=[1 1]  RectangleSizeUnits=m  BrickDimensions=[1 1 1]  BrickDimensionUnits=m  CylinderRadius=1  CylinderRadiusUnits=m  CylinderLength=1  CylinderLengthUnits=m  SphereRadius=1  SphereRadiusUnits=m  EllipsoidRadii=[1 1 1]  EllipsoidRadiiUnits=m  ExtrusionCrossSection=[1 1; -1 1; -1 -1; 1 -1]  ExtrusionCrossSectionUnits=m  ExtrusionLength=1  ExtrusionLengthUnits=m  PolygonNumSides=3  PolygonOuterRadius=1  PolygonOuterRadiusUnits=m  ExtGeomFileType=STL  ExtGeomFileName=geometry/flap.stl  ExtGeomFileUnits=m  RevolutionCrossSection=[1 1; 1 -1; 2 -1; 2 1]  RevolutionCrossSectionUnits=m  RevolutionExtent=Full  RevolutionAngle=180  RevolutionAngleUnits=deg  BlockFunction=simmechanics.library.body_elements.solid
  Bus Creator : BusCreator  Inputs=3
  External Force and Torque : sm_lib/Forces and Torques/External Force and Torque  ForceResolutionFrame=World  EnableForceX=off  EnableForceY=off  EnableForceZ=off  EnableForce=on  TorqueResolutionFrame=World  EnableTorqueX=off  EnableTorqueY=off  EnableTorqueZ=off  EnableTorque=on  BlockFunction=simmechanics.library.forces_torques.external_force_torque
  Motion Sensor: Stucture Response : Subsystem
  Selector : Selector  InputPortWidth=6  Indices=[1:3]
  Selector1 : Selector  InputPortWidth=6  Indices=[4:6]
  Setup CG : sm_lib/Frames and Transforms/Rigid Transform  TranslationMethod=Cartesian  TranslationLengthUnit=m  TranslationStandardAxis=+Z  TranslationStandardOffset=0  TranslationCartesianOffset=body.cg  TranslationROffset=0  TranslationROffsetUnits=m  TranslationZOffset=0  TranslationZOffsetUnits=m  TranslationThetaOffset=0  TranslationThetaOffsetUnits=deg  RotationMethod=None  RotationAngleUnits=rad  RotationStandardAxis=+Y  RotationAngle=0.05  RotationArbitraryAxis=[0.57735026918962584 0.57735026918962584 0.57735026918962584]  FollAlignAxisA=+X  BaseAlignAxisA=+Y  FollAlignAxisB=+Y  BaseAlignAxisB=+Z  BlockFunction=simmechanics.library.frames_transforms.rigid_transform
  Setup Initial Disp : sm_lib/Frames and Transforms/Rigid Transform  TranslationMethod=Cartesian  TranslationLengthUnit=m  TranslationStandardAxis=+Z  TranslationStandardOffset=0  TranslationCartesianOffset=body.initLinDisp  TranslationROffset=0  TranslationROffsetUnits=m  TranslationZOffset=0  TranslationZOffsetUnits=m  TranslationThetaOffset=0  TranslationThetaOffsetUnits=deg  RotationMethod=ArbitraryAxis  RotationAngleUnits=rad  RotationStandardAxis=+Y  RotationAngle=body.initAngularDispAngle  RotationArbitraryAxis=body.initAngularDispAxis  FollAlignAxisA=+X  BaseAlignAxisA=+Y  FollAlignAxisB=+Y  BaseAlignAxisB=+Z  BlockFunction=simmechanics.library.frames_transforms.rigid_transform
  Simulink-PS Converter1 : nesl_utility/Simulink-PS Converter  PhysicalDomain=network_engine_domain  SubClassName=ps_input  LeftPortType=input  RightPortType=output  PseudoPeriodic=off  Frequencies=[]  NoiseDistribution=none  NoiseParameters=[]  Unit=1  AffineConversion=off  InputFiltering=off  SimscapeFilterOrder=1  InputFilterTimeConstant=0.001  UdotUserProvided=1
  Simulink-PS Converter2 : nesl_utility/Simulink-PS Converter  PhysicalDomain=network_engine_domain  SubClassName=ps_input  LeftPortType=input  RightPortType=output  PseudoPeriodic=off  Frequencies=[]  NoiseDistribution=none  NoiseParameters=[]  Unit=1  AffineConversion=off  InputFiltering=off  SimscapeFilterOrder=1  InputFilterTimeConstant=0.001  UdotUserProvided=1
  World Frame : sm_lib/Frames and Transforms/World Frame  BlockFunction=simmechanics.library.frames_transforms.world_frame
  Connection(MFS) : PMIOPort  Port=1  Side=Right
  Response : Outport
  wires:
  F_vector/1 -> Selector1/1, Selector/1
  Selector/1 -> Simulink-PS Converter1/1
  Selector1/1 -> Simulink-PS Converter2/1
  Bus Creator/1 -> Response/1  "response"
  Motion Sensor: Stucture Response/1(Displacement) -> Bus Creator/1  "disp"
  Motion Sensor: Stucture Response/2(Velocity) -> Bus Creator/2  "vel"
  Motion Sensor: Stucture Response/3(Acceleration) -> Bus Creator/3  "accel"
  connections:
  Simulink-PS Converter1/RConn1 -- External Force and Torque/LConn1
  Simulink-PS Converter2/RConn1 -- External Force and Torque/LConn2
  Setup CG/LConn1 -- Connection(MFS)/RConn1
  Setup Initial Disp/LConn1 -- Setup CG/RConn1
  World Frame/RConn1 -- Motion Sensor: Stucture Response/LConn1
  Setup Initial Disp/RConn1 -- Body Properties/RConn1 -- External Force and Torque/RConn1 -- Body CG/RConn1 -- Motion Sensor: Stucture Response/RConn1

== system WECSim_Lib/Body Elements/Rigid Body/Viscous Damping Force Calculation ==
  Velocity : Inport
  Abs : Abs
  Times : Product  Inputs=**
  Viscous Damping : Gain  Gain=body.hydroForce.visDampingCoef  Multiplication=Matrix(K*u)
  F_Viscous : Outport
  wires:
  Velocity/1 -> Abs/1, Times/1
  Abs/1 -> Times/2
  Times/1 -> Viscous Damping/1
  Viscous Damping/1 -> F_Viscous/1  "F_Viscous"

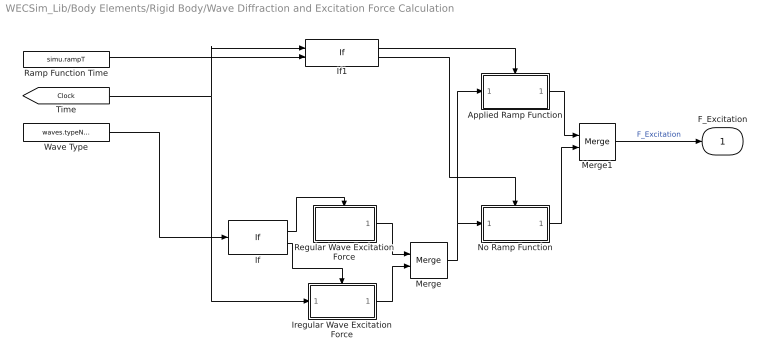
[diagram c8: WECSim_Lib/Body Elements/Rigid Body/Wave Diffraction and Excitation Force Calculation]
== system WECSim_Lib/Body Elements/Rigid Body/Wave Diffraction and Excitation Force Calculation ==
  Applied Ramp Function : Subsystem  TreatAsAtomicUnit=on
  If : If  IfExpression=u1 < 20
  If1 : If  NumInputs=2  IfExpression=u1 < u2
  Iregular Wave Excitation Force : Subsystem  TreatAsAtomicUnit=on
  Merge : Merge
  Merge1 : Merge
  No Ramp Function : Subsystem  TreatAsAtomicUnit=on
  Ramp Function Time : Constant  Value=simu.rampT
  Regular Wave Excitation Force : Subsystem  TreatAsAtomicUnit=on
  Wave Type : Constant  Value=waves.typeNum
  F_Excitation : Outport
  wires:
  [Clock] -> Iregular Wave Excitation Force/1(Time), If1/1
  Merge1/1 -> F_Excitation/1  "F_Excitation"
  No Ramp Function/1(Out1) -> Merge1/2
  Applied Ramp Function/1(Out1) -> Merge1/1
  If1/1 -> Applied Ramp Function/Action
  If1/2 -> No Ramp Function/Action
  Merge/1 -> Applied Ramp Function/1(In1), No Ramp Function/1(In1)
  Ramp Function Time/1 -> If1/2
  Iregular Wave Excitation Force/1(F_wave) -> Merge/2
  Regular Wave Excitation Force/1(F_wave) -> Merge/1
  If/2 -> Iregular Wave Excitation Force/Action
  If/1 -> Regular Wave Excitation Force/Action
  Wave Type/1 -> If/1

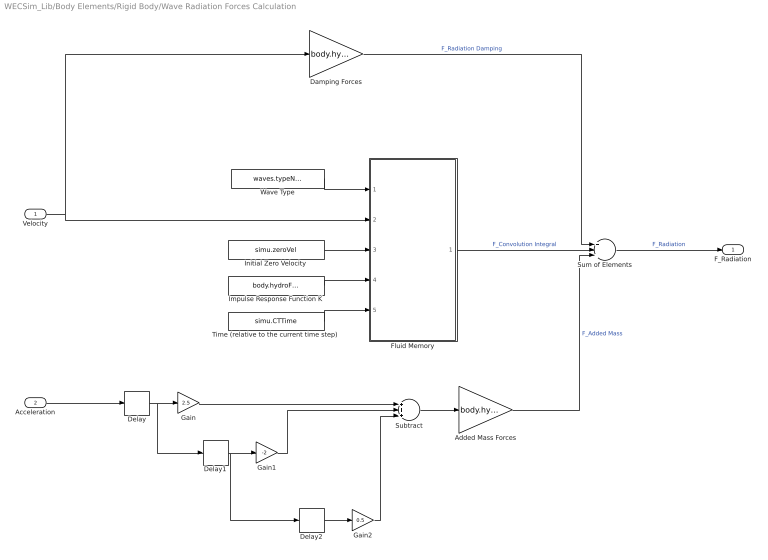
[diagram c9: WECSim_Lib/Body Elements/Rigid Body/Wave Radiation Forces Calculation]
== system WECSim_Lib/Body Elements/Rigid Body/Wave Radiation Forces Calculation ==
  Velocity : Inport
  Acceleration : Inport  Port=2
  Added Mass Forces : Gain  Gain=body.hydroForce.fAddedMass  Multiplication=Matrix(K*u)
  Damping Forces : Gain  Gain=body.hydroForce.fDamping  Multiplication=Matrix(K*u)
  Delay : Delay  DelayLength=1  InitialCondition=0
  Delay1 : Delay  DelayLength=1  InitialCondition=0
  Delay2 : Delay  DelayLength=1  InitialCondition=0
  Fluid Memory : MATLAB Function  TreatAsAtomicUnit=on
  Gain : Gain  Gain=2.5
  Gain1 : Gain  Gain=-2
  Gain2 : Gain  Gain=0.5
  Impulse Response Function K : Constant  Value=body.hydroForce.irkb
  Initial Zero Velocity : Constant  Value=simu.zeroVel
  Subtract : Sum  Inputs=+++
  Sum of Elements : Sum  Inputs=+++
  Time (relative to the current time step) : Constant  Value=simu.CTTime
  Wave Type : Constant  Value=waves.typeNum
  F_Radiation : Outport
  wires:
  Fluid Memory/1(F_FM) -> Sum of Elements/2  "F_Convolution Integral"
  Added Mass Forces/1 -> Sum of Elements/3  "F_Added Mass"
  Damping Forces/1 -> Sum of Elements/1  "F_Radiation Damping"
  Velocity/1 -> Fluid Memory/2(v), Damping Forces/1
  Initial Zero Velocity/1 -> Fluid Memory/3(ZeroVel)
  Impulse Response Function K/1 -> Fluid Memory/4(IRKB)
  Time (relative to the current time step)/1 -> Fluid Memory/5(CTTime)
  Wave Type/1 -> Fluid Memory/1(check)
  Acceleration/1 -> Delay/1
  Delay/1 -> Delay1/1, Gain/1
  Gain/1 -> Subtract/1
  Delay1/1 -> Gain1/1, Delay2/1
  Subtract/1 -> Added Mass Forces/1
  Delay2/1 -> Gain2/1
  Gain1/1 -> Subtract/2
  Gain2/1 -> Subtract/3
  Sum of Elements/1 -> F_Radiation/1  "F_Radiation"

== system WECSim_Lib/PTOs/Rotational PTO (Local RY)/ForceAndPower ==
  Pos : Inport
  Vel : Inport  Port=2
  Add : Sum
  Calculate Power : Product  Inputs=**
  Calculate Power1 : Product  Inputs=**
  Calculate Power2 : Product  Inputs=**
  Math Function : Math  Operator=square
  PCC Damping Coefficient : Constant  Value=pto.c
  PCC Stiffness Coefficient : Constant  Value=pto.k
  Force/Torque : Outport
  Power : Outport  Port=2
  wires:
  PCC Damping Coefficient/1 -> Calculate Power/1, Calculate Power1/1
  Calculate Power/1 -> Power/1
  Vel/1 -> Math Function/1, Calculate Power1/2
  PCC Stiffness Coefficient/1 -> Calculate Power2/2
  Pos/1 -> Calculate Power2/1
  Add/1 -> Force/Torque/1
  Math Function/1 -> Calculate Power/2
  Calculate Power2/1 -> Add/1
  Calculate Power1/1 -> Add/2

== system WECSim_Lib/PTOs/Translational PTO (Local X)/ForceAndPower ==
  Pos : Inport
  Vel : Inport  Port=2
  Add : Sum
  Calculate Power : Product  Inputs=**
  Calculate Power1 : Product  Inputs=**
  Calculate Power2 : Product  Inputs=**
  Math Function : Math  Operator=square
  PCC Damping Coefficient : Constant  Value=pto.c
  PCC Stiffness Coefficient : Constant  Value=pto.k
  Force : Outport
  Power : Outport  Port=2
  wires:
  PCC Damping Coefficient/1 -> Calculate Power/1, Calculate Power1/1
  Calculate Power/1 -> Power/1
  Vel/1 -> Math Function/1, Calculate Power1/2
  PCC Stiffness Coefficient/1 -> Calculate Power2/2
  Pos/1 -> Calculate Power2/1
  Add/1 -> Force/1
  Math Function/1 -> Calculate Power/2
  Calculate Power2/1 -> Add/1
  Calculate Power1/1 -> Add/2

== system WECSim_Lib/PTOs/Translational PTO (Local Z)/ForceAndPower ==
  Pos : Inport
  Vel : Inport  Port=2
  Add : Sum
  Calculate Power : Product  Inputs=**
  Calculate Power1 : Product  Inputs=**
  Calculate Power2 : Product  Inputs=**
  Math Function : Math  Operator=square
  PCC Damping Coefficient : Constant  Value=pto.c
  PCC Stiffness Coefficient : Constant  Value=pto.k
  Force : Outport
  Power : Outport  Port=2
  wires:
  PCC Damping Coefficient/1 -> Calculate Power/1, Calculate Power1/1
  Calculate Power/1 -> Power/1
  Vel/1 -> Math Function/1, Calculate Power1/2
  PCC Stiffness Coefficient/1 -> Calculate Power2/2
  Pos/1 -> Calculate Power2/1
  Add/1 -> Force/1
  Math Function/1 -> Calculate Power/2
  Calculate Power2/1 -> Add/1
  Calculate Power1/1 -> Add/2
